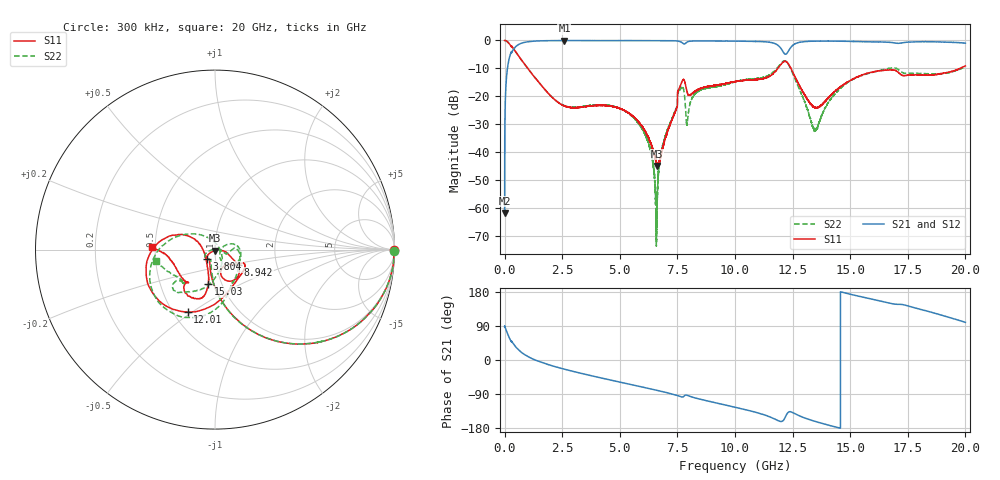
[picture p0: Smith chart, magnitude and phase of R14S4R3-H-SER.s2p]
!{R14S4R3}
!Johanson Technology Inc.
!www.johansontechnology.com
!Test Board Conditions:
!Substrate Type  RO4350B
!Substrate Thickness  20 mil
!Substrate Dk  3.66
!TL Type: GCPW
!TL Trace Width  36 mil
!TL Gap  12 mil
!Electrode orientation  Horizontal
!DUT TOPOLOGY	SERIES
!Mounting Pad LxW  26x36 mil
! Created Wed Nov 25 17:33:21 2020
! 2 Port Network Data from SP1.SP block
! freq  magS11  angS11  magS21  angS21  magS12  angS12  magS22  angS22
# khz S ma R 50
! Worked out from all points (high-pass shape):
!   20001 points, 300 kHz to 20 GHz, reference 50 ohm
!   highest |S21| = -0.03 dB at 2.596 GHz (marker M1); lowest = -61.7 dB at 300 kHz (marker M2)
!   |S21| within 3 dB of the highest: 395.9 MHz to 12.01 GHz (11.61 GHz wide, 187 % of centre); 12.38 GHz to end of sweep
!   lowest |S11| = -44.9 dB at 6.623 GHz (marker M3), VSWR 1.01, Z = 50 - j0.567 ohm
!   |S11| at or under -10 dB: 1.002 GHz to 11.86 GHz (10.86 GHz wide, 169 % of centre); 11.85937 GHz to 11.86092 GHz (1.549 MHz wide, 0.0131 % of centre); 12.43 GHz to 19.78 GHz (7.347 GHz wide, 45.6 % of centre)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
!   |S22| runs from -73.7 to 0.0 dB; largest |S21 - S12| = 0.02
!   S11 on the Smith chart (normalised r, x): 300 kHz: open; 3.804 GHz: 0.91, -0.09; 8.942 GHz: 1.27, -0.22; 12.01 GHz: 0.59, -0.48; 15.03 GHz: 0.87, -0.34; 20 GHz: 0.48, +0.02
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300  0.997 -0.2  0.0008177 87.7  0.0008271 90.6  0.9978 -0.3
113300  0.9547 -18.2  0.2934 71.7  0.2944 71.6  0.9551 -18.2
314300  0.7827 -40.9  0.6166 48.8  0.6177 48.8  0.7835 -40.9
1014300  0.3114 -80.6  0.9479 9.0  0.9485 9.0  0.312 -80.8
2596300  0.06728 -116.5  0.9964 -24.2  0.9948 -24.2  0.06788 -110.2
3334300  0.06381 -126.5  0.9939 -35.4  0.9944 -35.4  0.06508 -122.0
3804300  0.06793 -130.6  0.9938 -42.0  0.9948 -42.0  0.06909 -130.9
5784300  0.03594 -145.9  0.9943 -68.8  0.9937 -68.8  0.03376 -166.6
6290300  0.01619 -139.9  0.9925 -75.7  0.9943 -75.6  0.01211 -175.9
6623300  0.005677 -91.4  0.9938 -80.2  0.9936 -80.3  0.001397 9.8
6667300  0.006378 -69.9  0.9925 -80.9  0.9924 -80.8  0.003645 1.1
6867300  0.01201 -18.5  0.993 -83.7  0.9927 -83.7  0.01326 -4.2
7600300  0.1459 -32.4  0.9577 -95.7  0.9584 -95.8  0.1298 -2.4
7942300  0.1111 -70.1  0.9451 -93.4  0.9453 -93.4  0.03821 9.8
8942300  0.1538 -33.6  0.9803 -109.9  0.9792 -109.9  0.1451 -8.5
1.00003e7  0.1831 -25.6  0.9718 -124.5  0.972 -124.5  0.1815 -47.7
1.20103e7  0.3799 -113.6  0.7034 -162.3  0.7077 -162.2  0.3932 -106.4
1.25143e7  0.2674 163.8  0.8231 -138.8  0.8251 -139.1  0.251 166.8
1.33343e7  0.06958 177.0  0.9694 -159.4  0.9668 -159.3  0.03177 76.8
1.50253e7  0.1945 -100.7  0.9614 173.3  0.9632 173.0  0.1909 -98.8
1.66673e7  0.294 -114.7  0.9282 150.5  0.9208 150.3  0.3163 -130.7
2e7  0.3509 177.7  0.8944 99.4  0.8936 99.7  0.3373 -169.4
